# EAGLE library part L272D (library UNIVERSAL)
POWRE OP AMP
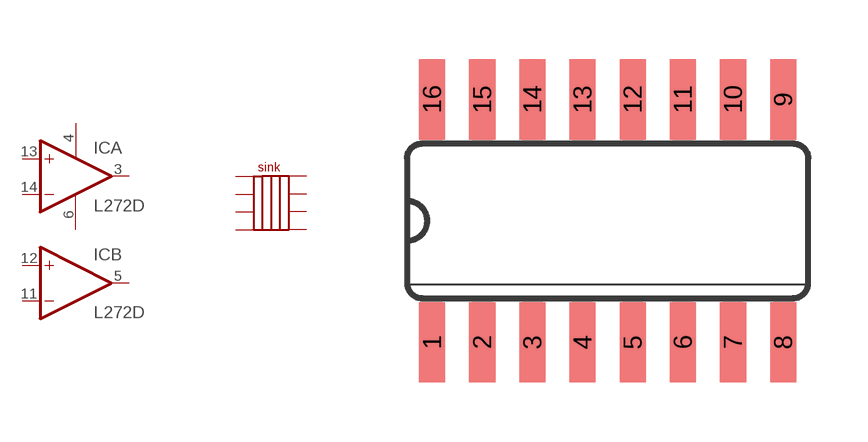
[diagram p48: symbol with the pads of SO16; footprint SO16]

Designator prefix IC; gates A=OPAMP B=OPAMP P=PWR+G G$4=SINK

## L272D  [SO16]
1  G$4:P$1
2  G$4:P$2
3  A:OUT  out
4  P:V+  pwr
5  B:OUT  out
6  P:GND  pwr
7  G$4:P$3
8  G$4:P$4
9  G$4:P$5
10  G$4:P$6
11  B:-IN  in
12  B:+IN  in
13  A:+IN  in
14  A:-IN  in
15  G$4:P$7
16  G$4:P$8

## Footprint SO16 (pad centres in mm)
smd 0.66 x 2.032: 1 -4.445,-3.073; 2 -3.175,-3.073; 3 -1.905,-3.073; 4 -0.635,-3.073; 5 0.635,-3.073; 6 1.905,-3.073; 7 3.175,-3.073; 8 4.445,-3.073; 9 4.445,3.073; 10 3.175,3.073; 11 1.905,3.073; 12 0.635,3.073; 13 -0.635,3.073; 14 -1.905,3.073; 15 -3.175,3.073; 16 -4.445,3.073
